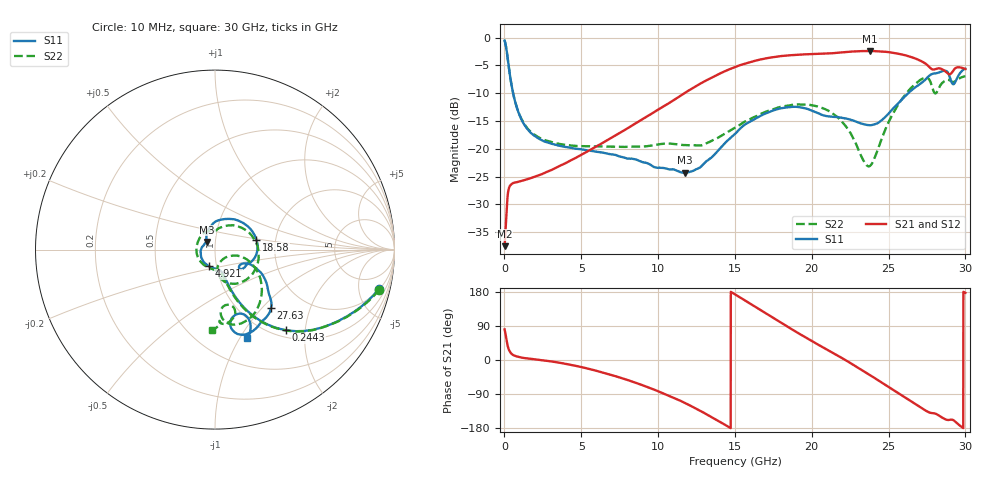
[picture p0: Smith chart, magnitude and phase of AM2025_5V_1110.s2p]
!Keysight Technologies,N5245B,MY58422270,A.16.20.02
!Date: Tuesday, July 14, 2026 01:15:08
!Correction: S11(C  2-Port  )
!S21(C  2-Port  )
!S12(C  2-Port  )
!S22(C  2-Port  )
!S2P File: Measurements: S11, S21, S12, S22:
# Hz S  dB  R 50
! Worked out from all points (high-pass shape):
!   3201 points, 10 MHz to 30 GHz, reference 50 ohm
!   highest |S21| = -2.41 dB at 23.81 GHz (marker M1); lowest = -37.5 dB at 10 MHz (marker M2)
!   |S21| within 3 dB of the highest: 14.91 GHz to 27.69 GHz (12.78 GHz wide, 60 % of centre); 29.41 GHz to 29.73 GHz (322 MHz wide, 1.09 % of centre)
!   lowest |S11| = -24.3 dB at 11.74 GHz (marker M3), VSWR 1.13, Z = 45.6 + j3.84 ohm
!   |S11| at or under -10 dB: 561.7 MHz to 26.29 GHz (25.73 GHz wide, 192 % of centre)
!   |S22| runs from -23.2 to -0.5 dB; largest |S21 - S12| = 0.01
!   S11 on the Smith chart (normalised r, x): 10 MHz: 2.13, -7.88; 244.3 MHz: 1.13, -1.58; 4.921 GHz: 0.92, -0.17; 18.58 GHz: 1.58, +0.18; 27.63 GHz: 1.37, -1.13; 30 GHz: 0.80, -1.08
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1e7  -0.55 -13.5  -37.53 80.8  -42.97 131.7  -0.52 -13.8
2.442969e8  -4.46 -48.6  -27.64 32.4  -27.64 31.8  -4.47 -48.9
5.910562e8  -10.37 -66.0  -26.14 12.6  -26.19 12.6  -10.35 -66.7
1.537616e9  -16.61 -71.2  -25.44 4.0  -25.43 4.0  -16.47 -73.7
4.920862e9  -20.08 -109.6  -21.21 -18.0  -21.21 -18.0  -19.53 -121.3
5.014581e9  -20.11 -111.2  -21.07 -18.8  -21.07 -18.9  -19.53 -123.1
1.000979e10  -23.43 159.8  -12.95 -82.6  -12.94 -82.5  -19.23 133.6
1.174359e10  -24.32 136.4  -9.95 -113.3  -9.95 -113.3  -19.35 99.5
1.34399e10  -21.66 125.5  -7.28 -149.6  -7.28 -149.6  -18.64 81.8
1.5005e10  -17.33 98.6  -5.31 173.3  -5.30 173.2  -16.22 60.7
1.659822e10  -14.18 60.5  -3.98 133.5  -3.98 133.4  -13.85 32.4
1.857568e10  -12.52 13.5  -3.19 84.1  -3.18 84.1  -12.19 -8.1
2.000958e10  -13.16 -15.0  -2.98 49.9  -2.98 49.9  -12.19 -37.4
2.208077e10  -14.49 -33.9  -2.64 2.4  -2.65 2.4  -15.49 -78.0
2.380519e10  -15.77 -33.2  -2.41 -40.2  -2.42 -40.2  -23.06 -43.4
2.500479e10  -13.67 -22.8  -2.62 -71.3  -2.63 -71.4  -15.19 -16.2
2.659801e10  -9.24 -33.4  -3.63 -112.9  -3.63 -112.9  -8.69 -45.5
2.762892e10  -6.91 -46.3  -5.24 -138.2  -5.24 -138.3  -7.48 -78.7
2.805065e10  -6.44 -55.8  -5.68 -141.6  -5.68 -141.8  -10.04 -78.0
2.900658e10  -7.30 -78.5  -6.60 -157.7  -6.59 -157.8  -7.75 -85.7
2.931585e10  -8.13 -66.4  -5.59 -161.7  -5.58 -161.7  -7.89 -86.0
3e10  -5.62 -69.8  -5.66 177.2  -5.61 177.0  -6.94 -92.4
